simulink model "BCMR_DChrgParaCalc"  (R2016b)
settings: Solver=FixedStepDiscrete  StartTime=0.0  StopTime=10  FixedStep=0.01  RelTol=1e-3  EnableMultiTasking=on
undefined symbols (not defined in the file or in its folder): BCMR_ahDChgBattNominalCapa_C, BCMR_bCurrCalSelect_C, BCMR_bCurrIncDeltaLimEna_C, BCMR_bDChrgFulChkTenEna_C, BCMR_bDChrgFulChkThreeEna_C, BCMR_cntCoolDFC_CW, BCMR_cntSoh_CW, BCMR_G1E0PlatformSwPara_C, BCMR_iCurrDcr_C, BCMR_iDcChrgCurrAbnorm_T, BCMR_iDcChrgCurrAbnormMAP_T, BCMR_iDcChrgCurrNew_T, BCMR_iDcChrgCurrNewMAP_T, BCMR_iDcChrgCurrOld_T, BCMR_iDcChrgCurrOldAbnorm_T, BCMR_iDcChrgCurrOldAbnormMAP_T, BCMR_iDcChrgCurrOldMAP_T, BCMR_iDCCurrDecStep_C, BCMR_iDCCurrDecThrd_C, BCMR_iDCCurrDeltaLim_C, BCMR_iDCCurrDiff_C, BCMR_iDCCurrFil_C, BCMR_iDCCurrIncStep_C, BCMR_iDCCurrIncThrd_C, BCMR_iDChrgCurrCutOff_C, BCMR_kmAcmDist_C, BCMR_numCcsPwrSelc_C, BCMR_numCellVoltFull_C, BCMR_numCellVoltFullThree_C, BCMR_numCurrCalcEna, BCMR_pCcsPwrSelc_C, BCMR_pctBmsPwrRdc_C, BCMR_rCurrDcr_C, BCMR_rCurrIcr_C, BCMR_rDchrgLoadCoef_C, BCMR_tBattTempMaxFil_C, BCMR_tBattTempSelcLmtDwn_C, BCMR_tBattTempSelcLmtUp_C, BCMR_tDcChrgCellTemp1_A, BCMR_tDcChrgCellTemp2_A, BCMR_tDcChrgCellTemp_A, BCMR_tDchrgLoadLmt_C, BCMR_tiBattTempMaxFilDly_C, BCMR_tiBattTempSwitch_C, BCMR_tiCellVoltFullCnt_C, BCMR_tiCellVoltMaxFilDly_C, BCMR_tiCurrHysTimeDelay_C, BCMR_tiDcChrgPwrCCSDebs_C, BCMR_tiDChgFullPreHold_C, BCMR_tiDChrgCurrReqCalDly_C, BCMR_tiDChrgDetParaDebs_C, BCMR_tiDChrgFullBase_C, BCMR_tiDChrgFullDebs_C, BCMR_tiDChrgFulParaDebs_C, BCMR_tiDChrgFulWait_C, BCMR_tiDChrgParaBase_C, BCMR_tiHoldOnToCurrCalcOff_C, BCMR_tTempDisMapX_A, BCMR_tTempDisMapY_A, BCMR_uBattVoltOff_C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
libraries: simulink x34
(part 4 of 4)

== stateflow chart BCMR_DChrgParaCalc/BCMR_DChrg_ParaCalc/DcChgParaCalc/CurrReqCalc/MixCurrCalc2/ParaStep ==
  state Init
    en:
    ParaStep = 0;
  state ParaStep1
    en:
    ParaStep = BCMR_ParaStep_A[0];
  state ParaStep2
    en:
    ParaStep = BCMR_ParaStep_A[1];
  state ParaStep3
    en:
    ParaStep = BCMR_ParaStep_A[2];
  state ParaStep4
    en:
    ParaStep = BCMR_ParaStep_A[3];
  state ParaStep5
    en:
    ParaStep = BCMR_ParaStep_A[4];
  state ParaStep6
    en:
    ParaStep = BCMR_ParaStep_A[5];
  state ParaStep7
    en:
    ParaStep = BCMR_ParaStep_A[6];
  state ParaStep8
    en:
    ParaStep = BCMR_ParaStep_A[7];
  state ParaStep9
    en:
    ParaStep = BCMR_ParaStep_A[8];
  state ParaStep10
    en:
    ParaStep = BCMR_ParaStep_A[9];
  state ParaStep11
    en:
    ParaStep = BCMR_ParaStep_A[10];
  state ParaStep12
    en:
    ParaStep = BCMR_ParaStep_A[11];
  state ParaStep13
    en:
    ParaStep = BCMR_ParaStep_A[12];
  state ParaStep14
    en:
    ParaStep = BCMR_ParaStep_A[13];
  (default) -> Init
  Init -> (junction 26) : [BattTemp >= BCMR_BattPara_A[0]]
  (junction 488) -> Init
  (junction 26) -> (junction 27)
  (junction 489) -> (junction 488)
  Init -> ParaStep1 : [BattTemp < BCMR_BattPara_A[0] && after(3,sec)]
  (junction 453) -> ParaStep1
  (junction 456) -> (junction 453)
  ParaStep1 -> ParaStep2 : [BattTemp >= BCMR_BattPara_A[0] && after(BCMR_tiCurrHysTimeDelay_C,sec) ]
  ParaStep2 -> (junction 456) : [BattTemp < BCMR_BattPara_A[0] ]
  (junction 27) -> ParaStep2
  (junction 447) -> (junction 456)
  (junction 27) -> (junction 28) : [BattTemp >= BCMR_BattPara_A[1] ]
  (junction 450) -> ParaStep2
  ParaStep2 -> ParaStep3 : [BattTemp >= BCMR_BattPara_A[1] && after(BCMR_tiCurrHysTimeDelay_C,sec) ]
  (junction 444) -> (junction 450)
  (junction 28) -> ParaStep3
  ParaStep3 -> (junction 444) : [BattTemp < BCMR_BattPara_A[1] - BCMR_HysRng_C]
  (junction 444) -> (junction 447) : [BattTemp < BCMR_BattPara_A[0] ]
  (junction 28) -> (junction 29) : [BattTemp >= BCMR_BattPara_A[2] ]
  (junction 430) -> (junction 444)
  (junction 431) -> (junction 447)
  (junction 441) -> ParaStep3
  (junction 426) -> (junction 441)
  ParaStep3 -> ParaStep4 : [BattTemp >= BCMR_BattPara_A[2] && after(BCMR_tiCurrHysTimeDelay_C,sec) ]
  ParaStep4 -> (junction 426) : [BattTemp < BCMR_BattPara_A[2] - BCMR_HysRng_C]
  (junction 426) -> (junction 430) : [BattTemp < BCMR_BattPara_A[1] - BCMR_HysRng_C]
  (junction 430) -> (junction 431) : [BattTemp < BCMR_BattPara_A[0] ]
  (junction 472) -> (junction 426)
  (junction 473) -> (junction 430)
  (junction 475) -> (junction 431)
  (junction 29) -> ParaStep4
  (junction 29) -> (junction 30) : [BattTemp >= BCMR_BattPara_A[3]]
  (junction 423) -> ParaStep4
  (junction 474) -> (junction 423)
  ParaStep4 -> ParaStep5 : [BattTemp >= BCMR_BattPara_A[3] && after(BCMR_tiCurrHysTimeDelay_C,sec)]
  ParaStep5 -> (junction 474) : [BattTemp < BCMR_BattPara_A[3] - BCMR_HysRng_C]
  (junction 474) -> (junction 472) : [BattTemp < BCMR_BattPara_A[2] - BCMR_HysRng_C]
  (junction 472) -> (junction 473) : [BattTemp < BCMR_BattPara_A[1] - BCMR_HysRng_C]
  (junction 473) -> (junction 475) : [BattTemp < BCMR_BattPara_A[0] ]
  (junction 30) -> ParaStep5
  (junction 401) -> (junction 474)
  (junction 389) -> (junction 472)
  (junction 400) -> (junction 473)
  (junction 398) -> (junction 475)
  (junction 30) -> (junction 31) : [BattTemp >= BCMR_BattPara_A[4] ]
  (junction 408) -> ParaStep5
  (junction 392) -> (junction 408)
  ParaStep5 -> ParaStep6 : [BattTemp >= BCMR_BattPara_A[4] && after(BCMR_tiCurrHysTimeDelay_C,sec) ]
  ParaStep6 -> (junction 392) : [BattTemp < BCMR_BattPara_A[4] - BCMR_HysRng_C]
  (junction 392) -> (junction 401) : [BattTemp < BCMR_BattPara_A[3] - BCMR_HysRng_C]
  (junction 401) -> (junction 389) : [BattTemp < BCMR_BattPara_A[2] - BCMR_HysRng_C]
  (junction 389) -> (junction 400) : [BattTemp < BCMR_BattPara_A[1] - BCMR_HysRng_C]
  (junction 400) -> (junction 398) : [BattTemp < BCMR_BattPara_A[0] ]
  (junction 375) -> (junction 392)
  (junction 371) -> (junction 401)
  (junction 364) -> (junction 389)
  (junction 369) -> (junction 400)
  (junction 376) -> (junction 398)
  (junction 31) -> ParaStep6
  (junction 31) -> (junction 74) : [BattTemp >= BCMR_BattPara_A[5] ]
  (junction 384) -> ParaStep6
  (junction 373) -> (junction 384)
  ParaStep6 -> ParaStep7 : [BattTemp >= BCMR_BattPara_A[5] && after(BCMR_tiCurrHysTimeDelay_C,sec) ]
  ParaStep7 -> (junction 373) : [BattTemp < BCMR_BattPara_A[5] - BCMR_HysRng_C]
  (junction 373) -> (junction 375) : [BattTemp < BCMR_BattPara_A[4] - BCMR_HysRng_C]
  (junction 375) -> (junction 371) : [BattTemp < BCMR_BattPara_A[3] - BCMR_HysRng_C]
  (junction 371) -> (junction 364) : [BattTemp < BCMR_BattPara_A[2] - BCMR_HysRng_C]
  (junction 364) -> (junction 369) : [BattTemp < BCMR_BattPara_A[1] - BCMR_HysRng_C]
  (junction 369) -> (junction 376) : [BattTemp < BCMR_BattPara_A[0]]
  (junction 341) -> (junction 373)
  (junction 349) -> (junction 375)
  (junction 352) -> (junction 371)
  (junction 343) -> (junction 364)
  (junction 353) -> (junction 369)
  (junction 350) -> (junction 376)
  (junction 74) -> ParaStep7
  (junction 74) -> (junction 75) : [BattTemp >= BCMR_BattPara_A[6] ]
  (junction 169) -> ParaStep7
  (junction 337) -> (junction 169)
  ParaStep7 -> ParaStep8 : [BattTemp >= BCMR_BattPara_A[6] && after(BCMR_tiCurrHysTimeDelay_C,sec) ]
  ParaStep8 -> (junction 337) : [BattTemp < BCMR_BattPara_A[6] - BCMR_HysRng_C]
  (junction 337) -> (junction 341) : [BattTemp < BCMR_BattPara_A[5] - BCMR_HysRng_C]
  (junction 341) -> (junction 349) : [BattTemp < BCMR_BattPara_A[4] - BCMR_HysRng_C]
  (junction 349) -> (junction 352) : [BattTemp < BCMR_BattPara_A[3] - BCMR_HysRng_C]
  (junction 352) -> (junction 343) : [BattTemp < BCMR_BattPara_A[2] - BCMR_HysRng_C]
  (junction 343) -> (junction 353) : [BattTemp < BCMR_BattPara_A[1] - BCMR_HysRng_C]
  (junction 353) -> (junction 350) : [BattTemp < BCMR_BattPara_A[0] ]
  (junction 75) -> ParaStep8
  (junction 313) -> (junction 337)
  (junction 321) -> (junction 341)
  (junction 328) -> (junction 349)
  (junction 331) -> (junction 352)
  (junction 319) -> (junction 343)
  (junction 334) -> (junction 353)
  (junction 330) -> (junction 350)
  (junction 75) -> (junction 76) : [BattTemp >= BCMR_BattPara_A[7] ]
  (junction 148) -> ParaStep8
  (junction 310) -> (junction 148)
  ParaStep8 -> ParaStep9 : [BattTemp >= BCMR_BattPara_A[7] && after(BCMR_tiCurrHysTimeDelay_C,sec) ]
  ParaStep9 -> (junction 310) : [BattTemp < BCMR_BattPara_A[7] - BCMR_HysRng_C]
  (junction 310) -> (junction 313) : [BattTemp < BCMR_BattPara_A[6] - BCMR_HysRng_C]
  (junction 313) -> (junction 321) : [BattTemp < BCMR_BattPara_A[5] - BCMR_HysRng_C]
  (junction 321) -> (junction 328) : [BattTemp < BCMR_BattPara_A[4] - BCMR_HysRng_C]
  (junction 328) -> (junction 331) : [BattTemp < BCMR_BattPara_A[3] - BCMR_HysRng_C]
  (junction 331) -> (junction 319) : [BattTemp < BCMR_BattPara_A[2] - BCMR_HysRng_C]
  (junction 319) -> (junction 334) : [BattTemp < BCMR_BattPara_A[1] - BCMR_HysRng_C]
  (junction 334) -> (junction 330) : [BattTemp < BCMR_BattPara_A[0]]
  (junction 280) -> (junction 310)
  (junction 283) -> (junction 313)
  (junction 299) -> (junction 321)
  (junction 295) -> (junction 328)
  (junction 293) -> (junction 331)
  (junction 287) -> (junction 319)
  (junction 290) -> (junction 334)
  (junction 292) -> (junction 330)
  (junction 76) -> ParaStep9
  (junction 76) -> (junction 77) : [BattTemp >= BCMR_BattPara_A[8] ]
  (junction 140) -> ParaStep9
  (junction 277) -> (junction 140)
  ParaStep9 -> ParaStep10 : [BattTemp >= BCMR_BattPara_A[8] && after(BCMR_tiCurrHysTimeDelay_C,sec) ]
  ParaStep10 -> (junction 277) : [BattTemp < BCMR_BattPara_A[8] - BCMR_HysRng_C]
  (junction 277) -> (junction 280) : [BattTemp < BCMR_BattPara_A[7] - BCMR_HysRng_C]
  (junction 280) -> (junction 283) : [BattTemp < BCMR_BattPara_A[6] - BCMR_HysRng_C]
  (junction 283) -> (junction 299) : [BattTemp < BCMR_BattPara_A[5] - BCMR_HysRng_C]
  (junction 299) -> (junction 295) : [BattTemp < BCMR_BattPara_A[4] - BCMR_HysRng_C]
  (junction 295) -> (junction 293) : [BattTemp < BCMR_BattPara_A[3] - BCMR_HysRng_C]
  (junction 293) -> (junction 287) : [BattTemp < BCMR_BattPara_A[2] - BCMR_HysRng_C]
  (junction 287) -> (junction 290) : [BattTemp < BCMR_BattPara_A[1] - BCMR_HysRng_C]
  (junction 290) -> (junction 292) : [BattTemp < BCMR_BattPara_A[0] ]
  (junction 228) -> (junction 277)
  (junction 230) -> (junction 280)
  (junction 232) -> (junction 283)
  (junction 247) -> (junction 299)
  (junction 253) -> (junction 295)
  (junction 249) -> (junction 293)
  (junction 259) -> (junction 287)
  (junction 256) -> (junction 290)
  (junction 246) -> (junction 292)
  (junction 77) -> ParaStep10
  (junction 77) -> (junction 78) : [BattTemp >= BCMR_BattPara_A[9] ]
  (junction 132) -> ParaStep10
  (junction 226) -> (junction 132)
  ParaStep10 -> ParaStep11 : [BattTemp >= BCMR_BattPara_A[9] && after(BCMR_tiCurrHysTimeDelay_C,sec) ]
  ParaStep11 -> (junction 226) : [BattTemp < BCMR_BattPara_A[9] - BCMR_HysRng_C]
  (junction 226) -> (junction 228) : [BattTemp < BCMR_BattPara_A[8] - BCMR_HysRng_C]
  (junction 228) -> (junction 230) : [BattTemp < BCMR_BattPara_A[7] - BCMR_HysRng_C]
  (junction 230) -> (junction 232) : [BattTemp < BCMR_BattPara_A[6] - BCMR_HysRng_C]
  (junction 232) -> (junction 247) : [BattTemp < BCMR_BattPara_A[5] - BCMR_HysRng_C]
  (junction 247) -> (junction 253) : [BattTemp < BCMR_BattPara_A[4] - BCMR_HysRng_C]
  (junction 253) -> (junction 249) : [BattTemp < BCMR_BattPara_A[3] - BCMR_HysRng_C]
  (junction 249) -> (junction 259) : [BattTemp < BCMR_BattPara_A[2] - BCMR_HysRng_C]
  (junction 259) -> (junction 256) : [BattTemp < BCMR_BattPara_A[1] - BCMR_HysRng_C]
  (junction 256) -> (junction 246) : [BattTemp < BCMR_BattPara_A[0] ]
  (junction 78) -> ParaStep11
  (junction 196) -> (junction 226)
  (junction 199) -> (junction 228)
  (junction 202) -> (junction 230)
  (junction 205) -> (junction 232)
  (junction 213) -> (junction 247)
  (junction 210) -> (junction 253)
  (junction 211) -> (junction 249)
  (junction 212) -> (junction 259)
  (junction 222) -> (junction 256)
  (junction 220) -> (junction 246)
  (junction 78) -> (junction 79) : [BattTemp >= BCMR_BattPara_A[10]]
  (junction 127) -> ParaStep11
  (junction 241) -> (junction 127)
  ParaStep11 -> ParaStep12 : [BattTemp >= BCMR_BattPara_A[10] && after(BCMR_tiCurrHysTimeDelay_C,sec)]
  ParaStep12 -> (junction 241) : [BattTemp < BCMR_BattPara_A[10] - BCMR_HysRng_C]
  (junction 241) -> (junction 196) : [BattTemp < BCMR_BattPara_A[9] - BCMR_HysRng_C]
  (junction 196) -> (junction 199) : [BattTemp < BCMR_BattPara_A[8] - BCMR_HysRng_C]
  (junction 199) -> (junction 202) : [BattTemp < BCMR_BattPara_A[7] - BCMR_HysRng_C]
  (junction 202) -> (junction 205) : [BattTemp < BCMR_BattPara_A[6] - BCMR_HysRng_C]
  (junction 205) -> (junction 213) : [BattTemp < BCMR_BattPara_A[5] - BCMR_HysRng_C]
  (junction 213) -> (junction 210) : [BattTemp < BCMR_BattPara_A[4] - BCMR_HysRng_C]
  (junction 210) -> (junction 211) : [BattTemp < BCMR_BattPara_A[3] - BCMR_HysRng_C]
  (junction 211) -> (junction 212) : [BattTemp < BCMR_BattPara_A[2] - BCMR_HysRng_C]
  (junction 212) -> (junction 222) : [BattTemp < BCMR_BattPara_A[1] - BCMR_HysRng_C]
  (junction 222) -> (junction 220) : [BattTemp < BCMR_BattPara_A[0] ]
  (junction 79) -> ParaStep12
  (junction 124) -> (junction 241)
  (junction 135) -> (junction 196)
  (junction 143) -> (junction 199)
  (junction 151) -> (junction 202)
  (junction 154) -> (junction 205)
  (junction 156) -> (junction 213)
  (junction 157) -> (junction 210)
  (junction 158) -> (junction 211)
  (junction 159) -> (junction 212)
  (junction 164) -> (junction 222)
  (junction 166) -> (junction 220)
  (junction 79) -> (junction 80) : [BattTemp >= BCMR_BattPara_A[11] ]
  (junction 119) -> ParaStep12
  (junction 238) -> (junction 119)
  ParaStep12 -> ParaStep13 : [BattTemp >= BCMR_BattPara_A[11] && after(BCMR_tiCurrHysTimeDelay_C,sec) ]
  (junction 80) -> ParaStep13
  ParaStep13 -> (junction 238) : [BattTemp < BCMR_BattPara_A[11] - BCMR_HysRng_C]
  (junction 238) -> (junction 124) : [BattTemp < BCMR_BattPara_A[10] - BCMR_HysRng_C]
  (junction 124) -> (junction 135) : [BattTemp < BCMR_BattPara_A[9] - BCMR_HysRng_C]
  (junction 135) -> (junction 143) : [BattTemp < BCMR_BattPara_A[8] - BCMR_HysRng_C]
  (junction 143) -> (junction 151) : [BattTemp < BCMR_BattPara_A[7] - BCMR_HysRng_C]
  (junction 151) -> (junction 154) : [BattTemp < BCMR_BattPara_A[6] - BCMR_HysRng_C]
  (junction 154) -> (junction 156) : [BattTemp < BCMR_BattPara_A[5] - BCMR_HysRng_C]
  (junction 156) -> (junction 157) : [BattTemp < BCMR_BattPara_A[4] - BCMR_HysRng_C]
  (junction 157) -> (junction 158) : [BattTemp < BCMR_BattPara_A[3] - BCMR_HysRng_C]
  (junction 158) -> (junction 159) : [BattTemp < BCMR_BattPara_A[2] - BCMR_HysRng_C]
  (junction 159) -> (junction 164) : [BattTemp < BCMR_BattPara_A[1] - BCMR_HysRng_C]
  (junction 164) -> (junction 166) : [BattTemp < BCMR_BattPara_A[0] ]
  (junction 80) -> (junction 81) : [BattTemp >= BCMR_BattPara_A[12] ]
  (junction 115) -> (junction 238)
  (junction 117) -> (junction 124)
  (junction 130) -> (junction 135)
  (junction 138) -> (junction 143)
  (junction 146) -> (junction 151)
  (junction 181) -> (junction 154)
  (junction 179) -> (junction 156)
  (junction 176) -> (junction 157)
  (junction 177) -> (junction 158)
  (junction 178) -> (junction 159)
  (junction 185) -> (junction 164)
  (junction 184) -> (junction 166) : [after(BCMR_tiDChrgFulWait_C,sec)]
  (junction 462) -> ParaStep13
  (junction 460) -> (junction 462)
  ParaStep13 -> ParaStep14 : [BattTemp >= BCMR_BattPara_A[12] && after(BCMR_tiCurrHysTimeDelay_C,sec) ]
  (junction 81) -> ParaStep14
  ParaStep14 -> (junction 460) : [BattTemp < BCMR_BattPara_A[12] - BCMR_HysRng_C]
  (junction 460) -> (junction 115) : [BattTemp < BCMR_BattPara_A[11] - BCMR_HysRng_C]
  (junction 115) -> (junction 117) : [BattTemp < BCMR_BattPara_A[10] - BCMR_HysRng_C]
  (junction 117) -> (junction 130) : [BattTemp < BCMR_BattPara_A[9] - BCMR_HysRng_C]
  (junction 130) -> (junction 138) : [BattTemp < BCMR_BattPara_A[8] - BCMR_HysRng_C]
  (junction 138) -> (junction 146) : [BattTemp < BCMR_BattPara_A[7] - BCMR_HysRng_C]
  (junction 146) -> (junction 181) : [BattTemp < BCMR_BattPara_A[6] - BCMR_HysRng_C]
  (junction 181) -> (junction 179) : [BattTemp < BCMR_BattPara_A[5] - BCMR_HysRng_C]
  (junction 179) -> (junction 176) : [BattTemp < BCMR_BattPara_A[4] - BCMR_HysRng_C]
  (junction 176) -> (junction 177) : [BattTemp < BCMR_BattPara_A[3] - BCMR_HysRng_C]
  (junction 177) -> (junction 178) : [BattTemp < BCMR_BattPara_A[2] - BCMR_HysRng_C]
  (junction 178) -> (junction 185) : [BattTemp < BCMR_BattPara_A[1] - BCMR_HysRng_C]
  (junction 185) -> (junction 184) : [BattTemp < BCMR_BattPara_A[0] ]
  (junction 81) -> (junction 467) : [BattTemp >= BCMR_BattPara_A[13] && after(BCMR_tiDChrgFulWait_C,sec)]
  ParaStep14 -> (junction 493) : [BattTemp >= BCMR_BattPara_A[13] && (after(BCMR_tiDChrgFulWait_C,sec) && BCMR_flgDChrgFulChk == true)]
  (junction 467) -> (junction 493)
  (junction 493) -> (junction 489)
  data: BattTemp input single; ParaStep output uint8; BCMR_BattPara_A input single; BCMR_ParaStep_A input uint8; BCMR_HysRng_C input single; BCMR_tiDChrgFulWait_C parameter single; BCMR_flgDChrgFulChk input boolean; BCMR_tiCurrHysTimeDelay_C parameter single

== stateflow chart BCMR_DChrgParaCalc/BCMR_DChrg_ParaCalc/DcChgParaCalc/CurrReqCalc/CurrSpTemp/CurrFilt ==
  state Init
    en:
    DCCurrReq=single(0);
  state Charging
    (default) -> (junction 10) : {DCCurrReq=single(0);}
    Charging -> (junction 10)
    (junction 10) -> (junction 13) : [DCChrgEn]
    (junction 10) -> (junction 48) : {DCCurrTarget=single(0); DCCurrReq=single(0);}
    (junction 13) -> (junction 23) : {DCCurrTarget=DCCurrReqIn; DeltaCurr=DCCurrTarget-DCCurrReq;}
    (junction 23) -> (junction 25) : [DeltaCurr<BCMR_iDCCurrDecThrd_C]
    (junction 23) -> (junction 27)
    (junction 25) -> (junction 34) : {DCCurrReq=max(DCCurrReq-BCMR_iDCCurrDecStep_C,DCCurrTarget);}
    (junction 27) -> (junction 29) : [DeltaCurr>BCMR_iDCCurrIncThrd_C]
    (junction 29) -> (junction 51) : [BCMR_bCurrIncDeltaLimEna_C]
    (junction 27) -> (junction 17) : {DCCurrReq=DCCurrTarget;}
    (junction 29) -> (junction 31) : {DCCurrReq=min(DCCurrReq+BCMR_iDCCurrIncStep_C,DCCurrTarget);}
    (junction 51) -> (junction 53) : {DCCurrReq=min(DCCurrReq+BCMR_iDCCurrIncStep_C,DCCurrTarget); DCCurrReq=min(DCCurrReq,BSPR_iBattCurr+BCMR_iDCCurrDeltaLim_C);}
    (junction 17) -> (junction 48)
    (junction 31) -> (junction 17)
    (junction 53) -> (junction 31)
    (junction 34) -> (junction 53)
  state ZeroCurr
    en:
    DCCurrReq=single(0);
  (default) -> Init
  Init -> Charging : [DCChrgEn]
  Charging -> ZeroCurr : [DCChrgStop]
  data: DCCurrReq output single; DCChrgEn input boolean; DCCurrReqIn input single; DCCurrTarget output single; DeltaCurr local single; BCMR_iDCCurrDecStep_C parameter single; BCMR_iDCCurrIncStep_C parameter single; DCChrgStop input boolean; BCMR_iDCCurrDecThrd_C parameter single; BCMR_iDCCurrIncThrd_C parameter single; BCMR_bCurrIncDeltaLimEna_C parameter boolean; BCMR_iDCCurrDeltaLim_C parameter double; BSPR_iBattCurr input single

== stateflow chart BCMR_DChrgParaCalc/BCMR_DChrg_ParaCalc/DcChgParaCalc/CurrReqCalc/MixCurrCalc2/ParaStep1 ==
  state Init
    en:
    ParaStep = 0;
  state ParaStep1
    en:
    ParaStep = BCMR_ParaStep_A[0];
  state ParaStep2
    en:
    ParaStep = BCMR_ParaStep_A[1];
  state ParaStep3
    en:
    ParaStep = BCMR_ParaStep_A[2];
  state ParaStep4
    en:
    ParaStep = BCMR_ParaStep_A[3];
  state ParaStep5
    en:
    ParaStep = BCMR_ParaStep_A[4];
  state ParaStep6
    en:
    ParaStep = BCMR_ParaStep_A[5];
  state ParaStep7
    en:
    ParaStep = BCMR_ParaStep_A[6];
  state ParaStep8
    en:
    ParaStep = BCMR_ParaStep_A[7];
  state ParaStep9
    en:
    ParaStep = BCMR_ParaStep_A[8];
  state ParaStep10
    en:
    ParaStep = BCMR_ParaStep_A[9];
  state ParaStep11
    en:
    ParaStep = BCMR_ParaStep_A[10];
  state ParaStep12
    en:
    ParaStep = BCMR_ParaStep_A[11];
  state ParaStep13
    en:
    ParaStep = BCMR_ParaStep_A[12];
  state ParaStep14
    en:
    ParaStep = BCMR_ParaStep_A[13];
  (default) -> Init
  Init -> (junction 26) : [BattTemp >= BCMR_BattPara_A[0]]
  (junction 488) -> Init
  (junction 26) -> (junction 27)
  (junction 489) -> (junction 488)
  Init -> ParaStep1 : [BattTemp < BCMR_BattPara_A[0]]
  (junction 453) -> ParaStep1
  (junction 456) -> (junction 453)
  ParaStep1 -> ParaStep2 : [BattTemp >= BCMR_BattPara_A[0] ]
  ParaStep2 -> (junction 456) : [BattTemp < BCMR_BattPara_A[0] ]
  (junction 27) -> ParaStep2
  (junction 447) -> (junction 456)
  (junction 27) -> (junction 28) : [BattTemp >= BCMR_BattPara_A[1] ]
  (junction 450) -> ParaStep2
  ParaStep2 -> ParaStep3 : [BattTemp >= BCMR_BattPara_A[1] ]
  (junction 444) -> (junction 450)
  (junction 28) -> ParaStep3
  ParaStep3 -> (junction 444) : [BattTemp < BCMR_BattPara_A[1] - BCMR_HysRng_C]
  (junction 444) -> (junction 447) : [BattTemp < BCMR_BattPara_A[0] ]
  (junction 28) -> (junction 29) : [BattTemp >= BCMR_BattPara_A[2] ]
  (junction 430) -> (junction 444)
  (junction 431) -> (junction 447)
  (junction 441) -> ParaStep3
  (junction 426) -> (junction 441)
  ParaStep3 -> ParaStep4 : [BattTemp >= BCMR_BattPara_A[2] ]
  ParaStep4 -> (junction 426) : [BattTemp < BCMR_BattPara_A[2] - BCMR_HysRng_C]
  (junction 426) -> (junction 430) : [BattTemp < BCMR_BattPara_A[1] - BCMR_HysRng_C]
  (junction 430) -> (junction 431) : [BattTemp < BCMR_BattPara_A[0] ]
  (junction 472) -> (junction 426)
  (junction 473) -> (junction 430)
  (junction 475) -> (junction 431)
  (junction 29) -> ParaStep4
  (junction 29) -> (junction 30) : [BattTemp >= BCMR_BattPara_A[3]]
  (junction 423) -> ParaStep4
  (junction 474) -> (junction 423)
  ParaStep4 -> ParaStep5 : [BattTemp >= BCMR_BattPara_A[3]]
  ParaStep5 -> (junction 474) : [BattTemp < BCMR_BattPara_A[3] - BCMR_HysRng_C]
  (junction 474) -> (junction 472) : [BattTemp < BCMR_BattPara_A[2] - BCMR_HysRng_C]
  (junction 472) -> (junction 473) : [BattTemp < BCMR_BattPara_A[1] - BCMR_HysRng_C]
  (junction 473) -> (junction 475) : [BattTemp < BCMR_BattPara_A[0] ]
  (junction 30) -> ParaStep5
  (junction 401) -> (junction 474)
  (junction 389) -> (junction 472)
  (junction 400) -> (junction 473)
  (junction 398) -> (junction 475)
  (junction 30) -> (junction 31) : [BattTemp >= BCMR_BattPara_A[4] ]
  (junction 408) -> ParaStep5
  (junction 392) -> (junction 408)
  ParaStep5 -> ParaStep6 : [BattTemp >= BCMR_BattPara_A[4] ]
  ParaStep6 -> (junction 392) : [BattTemp < BCMR_BattPara_A[4] - BCMR_HysRng_C]
  (junction 392) -> (junction 401) : [BattTemp < BCMR_BattPara_A[3] - BCMR_HysRng_C]
  (junction 401) -> (junction 389) : [BattTemp < BCMR_BattPara_A[2] - BCMR_HysRng_C]
  (junction 389) -> (junction 400) : [BattTemp < BCMR_BattPara_A[1] - BCMR_HysRng_C]
  (junction 400) -> (junction 398) : [BattTemp < BCMR_BattPara_A[0] ]
  (junction 375) -> (junction 392)
  (junction 371) -> (junction 401)
  (junction 364) -> (junction 389)
  (junction 369) -> (junction 400)
  (junction 376) -> (junction 398)
  (junction 31) -> ParaStep6
  (junction 31) -> (junction 74) : [BattTemp >= BCMR_BattPara_A[5] ]
  (junction 384) -> ParaStep6
  (junction 373) -> (junction 384)
  ParaStep6 -> ParaStep7 : [BattTemp >= BCMR_BattPara_A[5] ]
  ParaStep7 -> (junction 373) : [BattTemp < BCMR_BattPara_A[5] - BCMR_HysRng_C]
  (junction 373) -> (junction 375) : [BattTemp < BCMR_BattPara_A[4] - BCMR_HysRng_C]
  (junction 375) -> (junction 371) : [BattTemp < BCMR_BattPara_A[3] - BCMR_HysRng_C]
  (junction 371) -> (junction 364) : [BattTemp < BCMR_BattPara_A[2] - BCMR_HysRng_C]
  (junction 364) -> (junction 369) : [BattTemp < BCMR_BattPara_A[1] - BCMR_HysRng_C]
  (junction 369) -> (junction 376) : [BattTemp < BCMR_BattPara_A[0]]
  (junction 341) -> (junction 373)
  (junction 349) -> (junction 375)
  (junction 352) -> (junction 371)
  (junction 343) -> (junction 364)
  (junction 353) -> (junction 369)
  (junction 350) -> (junction 376)
  (junction 74) -> ParaStep7
  (junction 74) -> (junction 75) : [BattTemp >= BCMR_BattPara_A[6] ]
  (junction 169) -> ParaStep7
  (junction 337) -> (junction 169)
  ParaStep7 -> ParaStep8 : [BattTemp >= BCMR_BattPara_A[6] ]
  ParaStep8 -> (junction 337) : [BattTemp < BCMR_BattPara_A[6] - BCMR_HysRng_C]
  (junction 337) -> (junction 341) : [BattTemp < BCMR_BattPara_A[5] - BCMR_HysRng_C]
  (junction 341) -> (junction 349) : [BattTemp < BCMR_BattPara_A[4] - BCMR_HysRng_C]
  (junction 349) -> (junction 352) : [BattTemp < BCMR_BattPara_A[3] - BCMR_HysRng_C]
  (junction 352) -> (junction 343) : [BattTemp < BCMR_BattPara_A[2] - BCMR_HysRng_C]
  (junction 343) -> (junction 353) : [BattTemp < BCMR_BattPara_A[1] - BCMR_HysRng_C]
  (junction 353) -> (junction 350) : [BattTemp < BCMR_BattPara_A[0] ]
  (junction 75) -> ParaStep8
  (junction 313) -> (junction 337)
  (junction 321) -> (junction 341)
  (junction 328) -> (junction 349)
  (junction 331) -> (junction 352)
  (junction 319) -> (junction 343)
  (junction 334) -> (junction 353)
  (junction 330) -> (junction 350)
  (junction 75) -> (junction 76) : [BattTemp >= BCMR_BattPara_A[7] ]
  (junction 148) -> ParaStep8
  (junction 310) -> (junction 148)
  ParaStep8 -> ParaStep9 : [BattTemp >= BCMR_BattPara_A[7] ]
  ParaStep9 -> (junction 310) : [BattTemp < BCMR_BattPara_A[7] - BCMR_HysRng_C]
  (junction 310) -> (junction 313) : [BattTemp < BCMR_BattPara_A[6] - BCMR_HysRng_C]
  (junction 313) -> (junction 321) : [BattTemp < BCMR_BattPara_A[5] - BCMR_HysRng_C]
  (junction 321) -> (junction 328) : [BattTemp < BCMR_BattPara_A[4] - BCMR_HysRng_C]
  (junction 328) -> (junction 331) : [BattTemp < BCMR_BattPara_A[3] - BCMR_HysRng_C]
  (junction 331) -> (junction 319) : [BattTemp < BCMR_BattPara_A[2] - BCMR_HysRng_C]
  (junction 319) -> (junction 334) : [BattTemp < BCMR_BattPara_A[1] - BCMR_HysRng_C]
  (junction 334) -> (junction 330) : [BattTemp < BCMR_BattPara_A[0]]
  (junction 280) -> (junction 310)
  (junction 283) -> (junction 313)
  (junction 299) -> (junction 321)
  (junction 295) -> (junction 328)
  (junction 293) -> (junction 331)
  (junction 287) -> (junction 319)
  (junction 290) -> (junction 334)
  (junction 292) -> (junction 330)
  (junction 76) -> ParaStep9
  (junction 76) -> (junction 77) : [BattTemp >= BCMR_BattPara_A[8] ]
  (junction 140) -> ParaStep9
  (junction 277) -> (junction 140)
  ParaStep9 -> ParaStep10 : [BattTemp >= BCMR_BattPara_A[8] ]
  ParaStep10 -> (junction 277) : [BattTemp < BCMR_BattPara_A[8] - BCMR_HysRng_C]
  (junction 277) -> (junction 280) : [BattTemp < BCMR_BattPara_A[7] - BCMR_HysRng_C]
  (junction 280) -> (junction 283) : [BattTemp < BCMR_BattPara_A[6] - BCMR_HysRng_C]
  (junction 283) -> (junction 299) : [BattTemp < BCMR_BattPara_A[5] - BCMR_HysRng_C]
  (junction 299) -> (junction 295) : [BattTemp < BCMR_BattPara_A[4] - BCMR_HysRng_C]
  (junction 295) -> (junction 293) : [BattTemp < BCMR_BattPara_A[3] - BCMR_HysRng_C]
  (junction 293) -> (junction 287) : [BattTemp < BCMR_BattPara_A[2] - BCMR_HysRng_C]
  (junction 287) -> (junction 290) : [BattTemp < BCMR_BattPara_A[1] - BCMR_HysRng_C]
  (junction 290) -> (junction 292) : [BattTemp < BCMR_BattPara_A[0] ]
  (junction 228) -> (junction 277)
  (junction 230) -> (junction 280)
  (junction 232) -> (junction 283)
  (junction 247) -> (junction 299)
  (junction 253) -> (junction 295)
  (junction 249) -> (junction 293)
  (junction 259) -> (junction 287)
  (junction 256) -> (junction 290)
  (junction 246) -> (junction 292)
  (junction 77) -> ParaStep10
  (junction 77) -> (junction 78) : [BattTemp >= BCMR_BattPara_A[9] ]
  (junction 132) -> ParaStep10
  (junction 226) -> (junction 132)
  ParaStep10 -> ParaStep11 : [BattTemp >= BCMR_BattPara_A[9] ]
  ParaStep11 -> (junction 226) : [BattTemp < BCMR_BattPara_A[9] - BCMR_HysRng_C]
  (junction 226) -> (junction 228) : [BattTemp < BCMR_BattPara_A[8] - BCMR_HysRng_C]
  (junction 228) -> (junction 230) : [BattTemp < BCMR_BattPara_A[7] - BCMR_HysRng_C]
  (junction 230) -> (junction 232) : [BattTemp < BCMR_BattPara_A[6] - BCMR_HysRng_C]
  (junction 232) -> (junction 247) : [BattTemp < BCMR_BattPara_A[5] - BCMR_HysRng_C]
  (junction 247) -> (junction 253) : [BattTemp < BCMR_BattPara_A[4] - BCMR_HysRng_C]
  (junction 253) -> (junction 249) : [BattTemp < BCMR_BattPara_A[3] - BCMR_HysRng_C]
  (junction 249) -> (junction 259) : [BattTemp < BCMR_BattPara_A[2] - BCMR_HysRng_C]
  (junction 259) -> (junction 256) : [BattTemp < BCMR_BattPara_A[1] - BCMR_HysRng_C]
  (junction 256) -> (junction 246) : [BattTemp < BCMR_BattPara_A[0] ]
  (junction 78) -> ParaStep11
  (junction 196) -> (junction 226)
  (junction 199) -> (junction 228)
  (junction 202) -> (junction 230)
  (junction 205) -> (junction 232)
  (junction 213) -> (junction 247)
  (junction 210) -> (junction 253)
  (junction 211) -> (junction 249)
  (junction 212) -> (junction 259)
  (junction 222) -> (junction 256)
  (junction 220) -> (junction 246)
  (junction 78) -> (junction 79) : [BattTemp >= BCMR_BattPara_A[10]]
  (junction 127) -> ParaStep11
  (junction 241) -> (junction 127)
  ParaStep11 -> ParaStep12 : [BattTemp >= BCMR_BattPara_A[10]]
  ParaStep12 -> (junction 241) : [BattTemp < BCMR_BattPara_A[10] - BCMR_HysRng_C]
  (junction 241) -> (junction 196) : [BattTemp < BCMR_BattPara_A[9] - BCMR_HysRng_C]
  (junction 196) -> (junction 199) : [BattTemp < BCMR_BattPara_A[8] - BCMR_HysRng_C]
  (junction 199) -> (junction 202) : [BattTemp < BCMR_BattPara_A[7] - BCMR_HysRng_C]
  (junction 202) -> (junction 205) : [BattTemp < BCMR_BattPara_A[6] - BCMR_HysRng_C]
  (junction 205) -> (junction 213) : [BattTemp < BCMR_BattPara_A[5] - BCMR_HysRng_C]
  (junction 213) -> (junction 210) : [BattTemp < BCMR_BattPara_A[4] - BCMR_HysRng_C]
  (junction 210) -> (junction 211) : [BattTemp < BCMR_BattPara_A[3] - BCMR_HysRng_C]
  (junction 211) -> (junction 212) : [BattTemp < BCMR_BattPara_A[2] - BCMR_HysRng_C]
  (junction 212) -> (junction 222) : [BattTemp < BCMR_BattPara_A[1] - BCMR_HysRng_C]
  (junction 222) -> (junction 220) : [BattTemp < BCMR_BattPara_A[0] ]
  (junction 79) -> ParaStep12
  (junction 124) -> (junction 241)
  (junction 135) -> (junction 196)
  (junction 143) -> (junction 199)
  (junction 151) -> (junction 202)
  (junction 154) -> (junction 205)
  (junction 156) -> (junction 213)
  (junction 157) -> (junction 210)
  (junction 158) -> (junction 211)
  (junction 159) -> (junction 212)
  (junction 164) -> (junction 222)
  (junction 166) -> (junction 220)
  (junction 79) -> (junction 80) : [BattTemp >= BCMR_BattPara_A[11] ]
  (junction 119) -> ParaStep12
  (junction 238) -> (junction 119)
  ParaStep12 -> ParaStep13 : [BattTemp >= BCMR_BattPara_A[11] ]
  (junction 80) -> ParaStep13
  ParaStep13 -> (junction 238) : [BattTemp < BCMR_BattPara_A[11] - BCMR_HysRng_C]
  (junction 238) -> (junction 124) : [BattTemp < BCMR_BattPara_A[10] - BCMR_HysRng_C]
  (junction 124) -> (junction 135) : [BattTemp < BCMR_BattPara_A[9] - BCMR_HysRng_C]
  (junction 135) -> (junction 143) : [BattTemp < BCMR_BattPara_A[8] - BCMR_HysRng_C]
  (junction 143) -> (junction 151) : [BattTemp < BCMR_BattPara_A[7] - BCMR_HysRng_C]
  (junction 151) -> (junction 154) : [BattTemp < BCMR_BattPara_A[6] - BCMR_HysRng_C]
  (junction 154) -> (junction 156) : [BattTemp < BCMR_BattPara_A[5] - BCMR_HysRng_C]
  (junction 156) -> (junction 157) : [BattTemp < BCMR_BattPara_A[4] - BCMR_HysRng_C]
  (junction 157) -> (junction 158) : [BattTemp < BCMR_BattPara_A[3] - BCMR_HysRng_C]
  (junction 158) -> (junction 159) : [BattTemp < BCMR_BattPara_A[2] - BCMR_HysRng_C]
  (junction 159) -> (junction 164) : [BattTemp < BCMR_BattPara_A[1] - BCMR_HysRng_C]
  (junction 164) -> (junction 166) : [BattTemp < BCMR_BattPara_A[0] ]
  (junction 80) -> (junction 81) : [BattTemp >= BCMR_BattPara_A[12] ]
  (junction 115) -> (junction 238)
  (junction 117) -> (junction 124)
  (junction 130) -> (junction 135)
  (junction 138) -> (junction 143)
  (junction 146) -> (junction 151)
  (junction 181) -> (junction 154)
  (junction 179) -> (junction 156)
  (junction 176) -> (junction 157)
  (junction 177) -> (junction 158)
  (junction 178) -> (junction 159)
  (junction 185) -> (junction 164)
  (junction 184) -> (junction 166)
  (junction 462) -> ParaStep13
  (junction 460) -> (junction 462)
  ParaStep13 -> ParaStep14 : [BattTemp >= BCMR_BattPara_A[12] ]
  (junction 81) -> ParaStep14
  ParaStep14 -> (junction 460) : [BattTemp < BCMR_BattPara_A[12] - BCMR_HysRng_C]
  (junction 460) -> (junction 115) : [BattTemp < BCMR_BattPara_A[11] - BCMR_HysRng_C]
  (junction 115) -> (junction 117) : [BattTemp < BCMR_BattPara_A[10] - BCMR_HysRng_C]
  (junction 117) -> (junction 130) : [BattTemp < BCMR_BattPara_A[9] - BCMR_HysRng_C]
  (junction 130) -> (junction 138) : [BattTemp < BCMR_BattPara_A[8] - BCMR_HysRng_C]
  (junction 138) -> (junction 146) : [BattTemp < BCMR_BattPara_A[7] - BCMR_HysRng_C]
  (junction 146) -> (junction 181) : [BattTemp < BCMR_BattPara_A[6] - BCMR_HysRng_C]
  (junction 181) -> (junction 179) : [BattTemp < BCMR_BattPara_A[5] - BCMR_HysRng_C]
  (junction 179) -> (junction 176) : [BattTemp < BCMR_BattPara_A[4] - BCMR_HysRng_C]
  (junction 176) -> (junction 177) : [BattTemp < BCMR_BattPara_A[3] - BCMR_HysRng_C]
  (junction 177) -> (junction 178) : [BattTemp < BCMR_BattPara_A[2] - BCMR_HysRng_C]
  (junction 178) -> (junction 185) : [BattTemp < BCMR_BattPara_A[1] - BCMR_HysRng_C]
  (junction 185) -> (junction 184) : [BattTemp < BCMR_BattPara_A[0] ]
  (junction 81) -> (junction 467) : [BattTemp >= BCMR_BattPara_A[13] ]
  ParaStep14 -> (junction 493) : [BattTemp >= BCMR_BattPara_A[13] ]
  (junction 467) -> (junction 493)
  (junction 493) -> (junction 489)
  data: BattTemp input single; ParaStep output uint8; BCMR_BattPara_A input single; BCMR_ParaStep_A input uint8; BCMR_HysRng_C input single
